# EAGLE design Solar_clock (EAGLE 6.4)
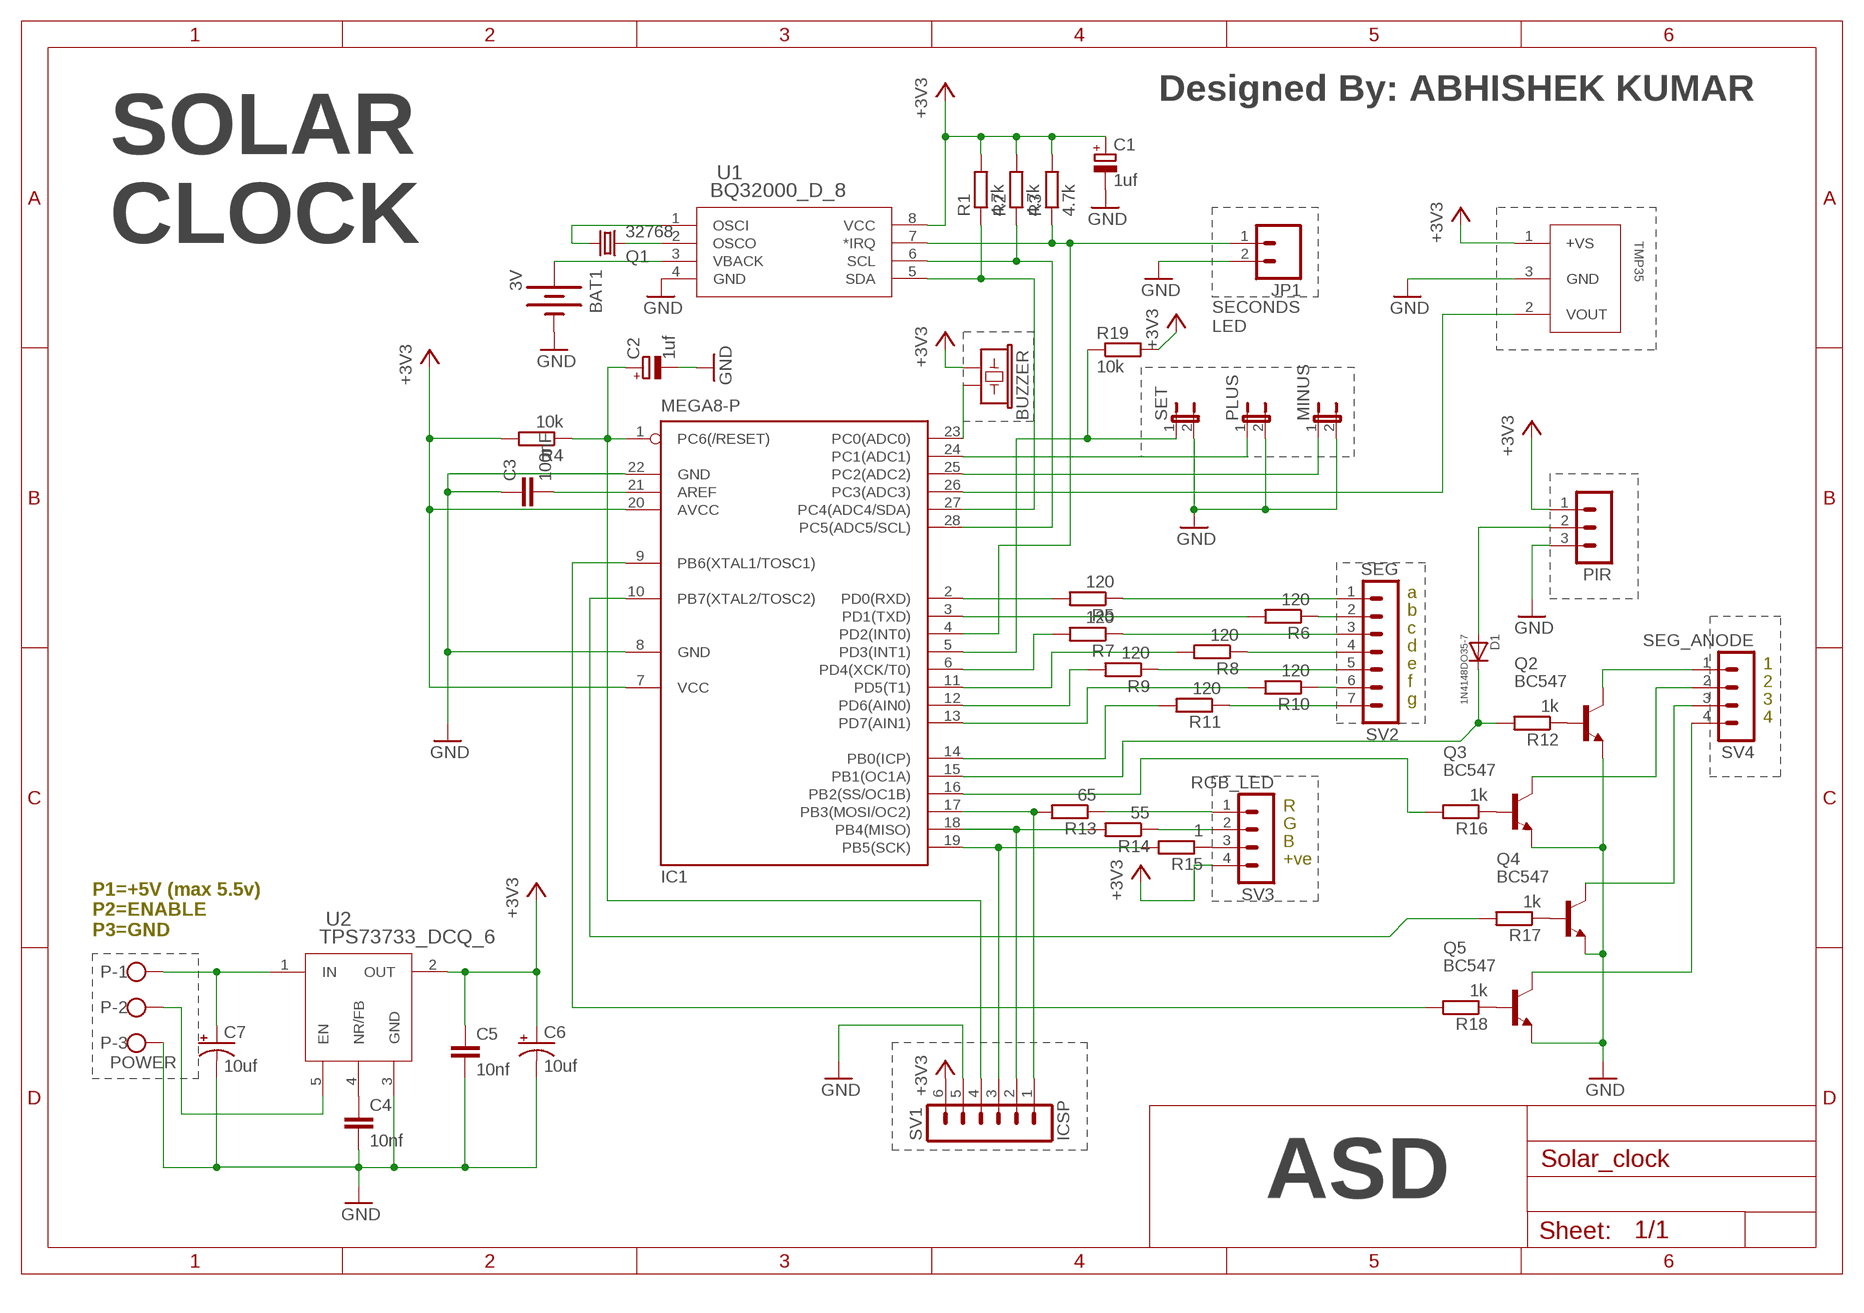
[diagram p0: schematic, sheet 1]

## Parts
BAT1  3V  BATTERY20PTH  [BATTCOM_20MM_PTH]
BUZZER  BUZZERNS  [BUZZER-12MM-NS]
C1  1uf  CPOL-EUE2.5-5  [E2,5-5]
C2  1uf  CPOL-EUE5-5  [E5-5]
C3  100nF  C-EU050-024X044  [C050-024X044]
C4  10nf  C-EU050-030X075  [C050-030X075]
C5  10nf  C-EU050-025X075  [C050-025X075]
C6  10uf  CPOL-USE2.5-6  [E2,5-6]
C7  10uf  CPOL-USE2.5-6  [E2,5-6]
D1  1N4148DO35-7  [DO35-7]
IC1  MEGA8-P  [DIL28-3]
JP1  M02PTH  [1X02]
MINUS  JUMPER-2PTH  [1X02]
P  POWER  W237-103  [W237-103]
PIR  MA03-1  [MA03-1]
PLUS  JUMPER-2PTH  [1X02]
Q1  32768  CRYSTALTC38H  [TC38H]
Q2  BC547  [TO92]
Q3  BC547  [TO92]
Q4  BC547  [TO92]
Q5  BC547  [TO92]
R1  4.7k  R-EU_R1206  [R1206]
R2  4.7k  R-EU_R1206  [R1206]
R3  4.7k  R-EU_R1206  [R1206]
R4  10k  R-EU_R1206  [R1206]
R5  120  R-EU_R1206  [R1206]
R6  120  R-EU_R1206  [R1206]
R7  120  R-EU_R1206  [R1206]
R8  120  R-EU_R1206  [R1206]
R9  120  R-EU_R1206  [R1206]
R10  120  R-EU_R1206  [R1206]
R11  120  R-EU_R1206  [R1206]
R12  1k  R-EU_R1206  [R1206]
R13  65  R-EU_R1206  [R1206]
R14  55  R-EU_R1206  [R1206]
R15  1  R-EU_R1206  [R1206]
R16  1k  R-EU_R1206  [R1206]
R17  1k  R-EU_R1206  [R1206]
R18  1k  R-EU_R1206  [R1206]
R19  10k  R-EU_R1206  [R1206]
SET  JUMPER-2PTH  [1X02]
SV1  ICSP  MA06-1  [MA06-1]
SV2  SEG  MA07-1  [MA07-1]
SV3  RGB_LED  MA04-1  [MA04-1]
SV4  SEG_ANODE  MA04-1  [MA04-1]
TMP35  TMP35GT9  [T_3]
U1  BQ32000_D_8  [D8]
U2  TPS73733_DCQ_6  [DCQ6]

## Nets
+3V3: BUZZER.+ C1.+ C5.1 C6.+ IC1.7(VCC) IC1.20(AVCC) PIR.1 R1.2 R2.2 R3.2 R4.2 R19.2 SV1.6 SV3.4 TMP35.1(+VS) U1.8(VCC) U2.2(OUT)
GND: BAT1.2(-) C1.- C2.- C3.1 C4.2 C5.2 C6.- C7.- IC1.8(GND) IC1.22(GND) JP1.2 MINUS.2 P.3 PIR.3 PLUS.2 Q2.1(E) Q3.1(E) Q4.1(E) Q5.1(E) SET.2 SV1.5 TMP35.3(GND) U1.4(GND) U2.3(GND)
N$1: IC1.28(PC5(ADC5/SCL)) R2.1 U1.6(SCL)
N$2: IC1.27(PC4(ADC4/SDA)) R1.1 U1.5(SDA)
N$3: IC1.4(PD2(INT0)) JP1.1 R3.1 U1.7(*IRQ)
N$4: Q1.2 U1.2(OSCO)
N$5: Q1.1 U1.1(OSCI)
N$6: C2.+ IC1.1(PC6(/RESET)) R4.1 SV1.4
N$7: C3.2 IC1.21(AREF)
N$8: IC1.17(PB3(MOSI/OC2)) R13.2 SV1.1
N$9: IC1.18(PB4(MISO)) R14.2 SV1.2
N$10: IC1.19(PB5(SCK)) R15.2 SV1.3
N$11: IC1.2(PD0(RXD)) R5.2
N$12: IC1.14(PB0(ICP)) R11.2
N$13: IC1.13(PD7(AIN1)) R10.2
N$14: IC1.6(PD4(XCK/T0)) R7.2
N$15: IC1.11(PD5(T1)) R8.2
N$16: R15.1 SV3.3
N$17: IC1.3(PD1(TXD)) R6.2
N$18: IC1.12(PD6(AIN0)) R9.2
N$19: IC1.5(PD3(INT1)) R19.1 SET.1
N$20: IC1.24(PC1(ADC1)) PLUS.1
N$21: IC1.25(PC2(ADC2)) MINUS.1
N$22: IC1.26(PC3(ADC3)) TMP35.2(VOUT)
N$23: BUZZER.- IC1.23(PC0(ADC0))
N$24: R5.1 SV2.1
N$25: R6.1 SV2.2
N$26: R7.1 SV2.3
N$27: R10.1 SV2.6
N$28: R9.1 SV2.5
N$29: R11.1 SV2.7
N$30: R8.1 SV2.4
N$31: R14.1 SV3.2
N$32: R13.1 SV3.1
N$33: Q2.2(B) R12.1
N$34: Q3.2(B) R16.1
N$35: Q4.2(B) R17.1
N$36: Q5.2(B) R18.1
N$37: Q3.3(C) SV4.2
N$38: Q5.3(C) SV4.4
N$39: Q4.3(C) SV4.3
N$40: Q2.3(C) SV4.1
N$41: D1.C IC1.15(PB1(OC1A)) R12.2
N$42: IC1.16(PB2(SS/OC1B)) R16.2
N$43: IC1.10(PB7(XTAL2/TOSC2)) R17.2
N$44: IC1.9(PB6(XTAL1/TOSC1)) R18.2
N$45: BAT1.1(+) U1.3(VBACK)
N$46: C4.1 U2.4(NR/FB)
N$47: C7.+ P.1 U2.1(IN)
N$48: P.2 U2.5(EN)
N$51: D1.A PIR.2

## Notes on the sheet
- Designed By: ABHISHEK KUMAR
- SOLAR
- CLOCK
- SECONDS
  LED
- a
- b
- c
- d
- e | 1
- f | 2
- g | 3
- 4
- R
- G
- B
- +ve
- P1=+5V (max 5.5v)
  P2=ENABLE
  P3=GND
- ASD

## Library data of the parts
BAT1 = SparkFun:BATTERY: Battery Holders
BUZZER = SparkFun:BUZZER: Buzzer 12mm
C1 C2 = resistor:CPOL-EU: POLARIZED CAPACITOR, European symbol
C3-C5 = resistor:C-EU: CAPACITOR, European symbol
C6 C7 = resistor:CPOL-US: POLARIZED CAPACITOR, American symbol
D1 = diode:1N4148: DIODE
IC1 = atmel:MEGA8-P: MICROCONTROLLER 8 Kbytes FLASH, 1 kbytes SRAM, 512 bytes EEPROM, USART, 4-channel 10 bit ADC, 2-channel 8 bit ADC Pin compatible with Atmega48, ATMega88, ATMega168 Source: avr.lbr; OC_FARNELL: unknown; OC_NEWARK: unknown
JP1 = SparkFun:M02: Header 2
MINUS PLUS SET = SparkFun:JUMPER-2: Jumper
P = con-wago-500:W237-103: WAGO SCREW CLAMP; MPN: 237-103; OC_FARNELL: unknown; OC_NEWARK: 18M7116
PIR = con-lstb:MA03-1: PIN HEADER; OC_FARNELL: unknown; OC_NEWARK: unknown
Q1 = SparkFun:CRYSTAL: Crystals
Q2-Q5 = transistor-npn:BC547*: NPN Transistor
R1-R19 = resistor:R-EU_: RESISTOR, European symbol
SV1 = con-lstb:MA06-1: PIN HEADER; OC_FARNELL: unknown; OC_NEWARK: unknown
SV2 = con-lstb:MA07-1: PIN HEADER; OC_FARNELL: unknown; OC_NEWARK: unknown
SV3 SV4 = con-lstb:MA04-1: PIN HEADER; OC_FARNELL: unknown; OC_NEWARK: unknown
TMP35 = TMP35:TMP35GT9; MANUFACTURER_PART_NUMBER: TMP35GT9; VENDOR: Vendor
U1 = BQ32000:BQ32000_D_8; DATASHEETURL: http://www.ti.com/lit/gpn/BQ32000; DESCRIPTION: Serial RTC with Battery Backup and Trickle Charge; FAMILY_NAME: REAL-TIME CLOCK; GENERIC_PART_NUMBER: BQ32000; INDUSTRY_STD_PKG_TYPE: SOIC; MANUFACTURER: Texas Instruments; PACKAGE_DESIGNATOR: D; PIN_COUNT: 8
U2 = TPS73733:TPS73733_DCQ_6; DATASHEETURL: http://www.ti.com/lit/gpn/TPS73733; DESCRIPTION: Single Output LDO, 1A, Fixed (3.3V), Reverse Current Protection; FAMILY_NAME: SINGLE CHANNEL LDO; GENERIC_PART_NUMBER: TPS73733; INDUSTRY_STD_PKG_TYPE: SOT-223; MANUFACTURER: Texas Instruments; MANUFACTURER_PART_NUMBER: tps73733_dcq_6; PACKAGE_DESIGNATOR: DCQ; PIN_COUNT: 6; VENDOR: Texas Instruments

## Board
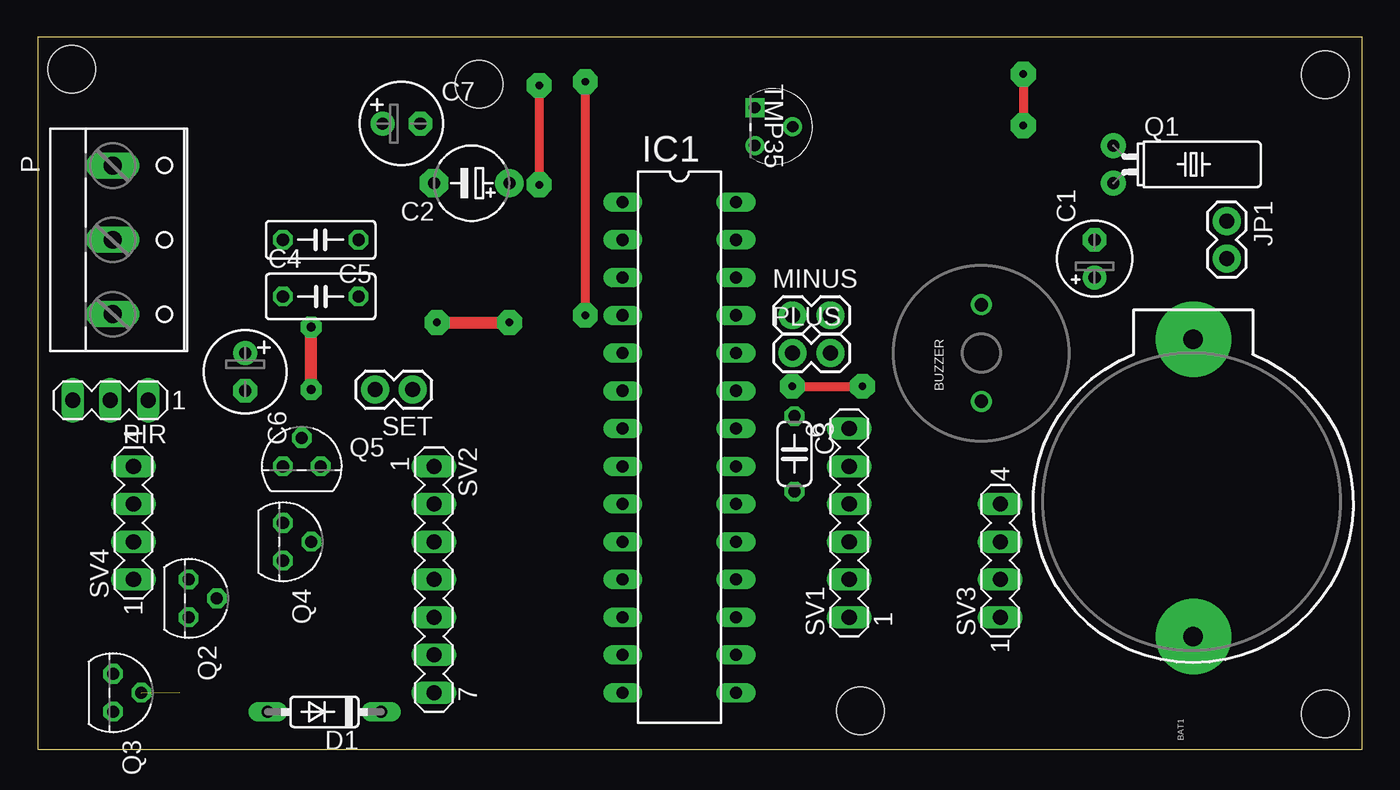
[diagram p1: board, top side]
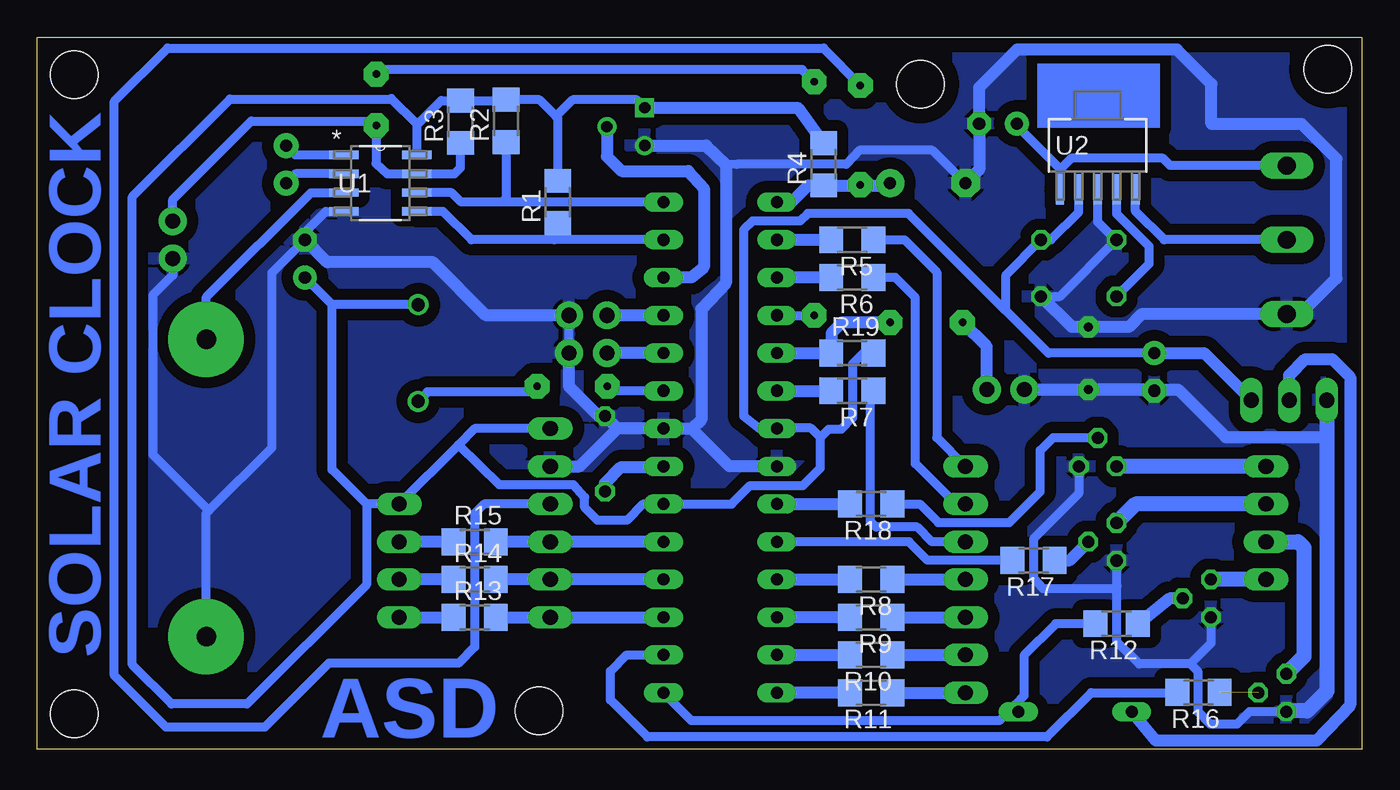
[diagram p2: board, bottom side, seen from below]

Size 89.13 x 47.93 mm. Coordinates in mm from the lower left corner, seen from the top.
Outline: 0,0 89.13,0 89.13,47.93 0,47.93 0,0
Copper layers (1*16): Top 0.035mm / dielectric 1.5mm / Bottom 0.035mm
Design rules "default *": minimum track width 10mil, minimum drill 24mil, track to track 30mil, track to pad 30mil, pad to pad 8mil, via to via 8mil, smd to smd 8mil, copper to edge 40mil, drill to drill 8mil, minimum pad ring 10mil, minimum via ring 8mil, stop-mask expansion 4mil, vias tented up to drill 0mil, thermal gap 10mil
Holes 3.2 mm at 86.64,45.42 86.64,2.39 29.72,44.75 2.29,45.77 55.37,2.59

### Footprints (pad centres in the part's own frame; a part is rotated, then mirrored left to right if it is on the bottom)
BATTCOM_20MM_PTH = drill 1.3: 1 20,0; 2 0,0
BUZZER-12MM-NS = drill 0.9: + 3.25,0; - -3.25,0
E2,5-5 = drill 0.813 pad 1.6: + -1.27,0 | drill 0.813 pad 1.6 octagon: - 1.27,0
E5-5 = drill 0.813 pad 1.905: + -2.54,0 | drill 0.813 pad 1.905 octagon: - 2.54,0
C050-024X044 = drill 0.813 octagon: 1 -2.54,0; 2 2.54,0
C050-030X075 = drill 0.813 octagon: 1 -2.54,0; 2 2.54,0
C050-025X075 = drill 0.813 octagon: 1 -2.54,0; 2 2.54,0
E2,5-6 = drill 0.813 pad 1.6: + -1.27,0 | drill 0.813 pad 1.6 octagon: - 1.27,0
DO35-7 = drill 0.813 long: A 3.81,0; C -3.81,0
DIL28-3 = drill 0.813 long: 1 -16.51,-3.81; 2 -13.97,-3.81; 3 -11.43,-3.81; 4 -8.89,-3.81; 5 -6.35,-3.81; 6 -3.81,-3.81; 7 -1.27,-3.81; 8 1.27,-3.81; 9 3.81,-3.81; 10 6.35,-3.81; 11 8.89,-3.81; 12 11.43,-3.81; 13 13.97,-3.81; 14 16.51,-3.81; 15 16.51,3.81; 16 13.97,3.81; 17 11.43,3.81; 18 8.89,3.81; 19 6.35,3.81; 20 3.81,3.81; 21 1.27,3.81; 22 -1.27,3.81; 23 -3.81,3.81; 24 -6.35,3.81; 25 -8.89,3.81; 26 -11.43,3.81; 27 -13.97,3.81; 28 -16.51,3.81
1X02 = drill 1.016 pad 1.88: 1 0,0; 2 2.54,0
W237-103 = drill 1.194 long: 1 -5,-1.29; 2 0,-1.29; 3 5,-1.29
MA03-1 = drill 1.016 long: 1 -2.54,0; 2 0,0; 3 2.54,0
TC38H = drill 0.813 pad 1.676: 1 -1.27,0; 2 1.27,0
TO92 = drill 0.813 octagon: 1 1.27,0; 2 0,1.905; 3 -1.27,0
R1206 = smd 1.6 x 1.803: 1 -1.422,0; 2 1.422,0
MA06-1 = drill 1.016 long: 1 -6.35,0; 2 -3.81,0; 3 -1.27,0; 4 1.27,0; 5 3.81,0; 6 6.35,0
MA07-1 = drill 1.016 long: 1 -7.62,0; 2 -5.08,0; 3 -2.54,0; 4 0,0; 5 2.54,0; 6 5.08,0; 7 7.62,0
MA04-1 = drill 1.016 long: 1 -3.81,0; 2 -1.27,0; 3 1.27,0; 4 3.81,0
T_3 = drill 0.762 square: 1 -2.54,-2.54 | drill 0.762: 2 -1.27,0; 3 0,-2.54
D8 = smd 1.981 x 0.559: 1 -2.464,1.905; 2 -2.464,0.635; 3 -2.464,-0.635; 4 -2.464,-1.905; 5 2.464,-1.905; 6 2.464,-0.635; 7 2.464,0.635; 8 2.464,1.905
DCQ6 = smd 0.559 x 2.057: 1 -2.54,-2.946; 2 -1.27,-2.946; 3 0,-2.946; 4 1.27,-2.946; 5 2.54,-2.946

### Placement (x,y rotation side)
BAT1  77.75,7.59 90 top
BUZZER  63.5,26.67 90 top
C1  71.12,33.02 90 top
C2  29.21,38.1 180 top
C3  50.93,19.89 270 top
C4  19.05,30.48 0 top
C5  19.05,34.29 180 top
C6  13.97,25.4 270 top
C7  24.49,42.11 0 top
D1  19.3,2.51 180 top
IC1  43.18,20.32 270 top
JP1  80.01,35.56 270 top
MINUS  50.8,29.21 0 top
P  6.35,34.29 270 top
PIR  4.9,23.5 180 top
PLUS  50.8,26.67 0 top
Q1  72.39,39.37 270 top
Q2  10.16,10.16 270 top
Q3  5.08,3.81 270 top
Q4  16.51,13.97 270 top
Q5  17.78,19.05 0 top
R1  54.1,36.83 90 bottom
R2  57.58,42.29 90 bottom
R3  60.66,42.24 90 bottom
R4  36.22,39.37 90 bottom
R5  34.29,34.29 180 bottom
R6  34.29,31.75 180 bottom
R7  34.29,24.13 180 bottom
R8  33.02,11.43 180 bottom
R9  33.02,8.89 180 bottom
R10  33.02,6.35 180 bottom
R11  33.02,3.81 180 bottom
R12  16.51,8.46 180 bottom
R13  59.69,8.89 0 bottom
R14  59.69,11.43 0 bottom
R15  59.69,13.97 0 bottom
R16  11,3.84 180 bottom
R17  22.1,12.73 180 bottom
R18  33.02,16.51 180 bottom
R19  34.29,26.67 0 bottom
SET  25.25,24.21 180 top
SV1  54.61,15.24 90 top
SV2  26.67,11.43 270 top
SV3  64.77,12.7 90 top
SV4  6.45,15.24 90 top
TMP35  50.8,40.64 270 top
U1  66.04,38.1 0 bottom
U2  17.78,40.64 0 bottom

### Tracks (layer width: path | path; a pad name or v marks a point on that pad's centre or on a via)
+3V3
  Bottom 0.61: TMP35.1 48.79,43.71 53.11,43.71 54.23,42.6 | R1.2 54.1,42.47 54.23,42.6 | 54.23,42.6 55.35,43.71 R2.2 57.63,43.66 R3.2 61.95,43.66 63.58,42.04 U1.8 63.58,42.06 65.3,43.79 65.33,43.76 76.15,43.76 82.73,37.19 82.73,5.69 80.09,3.05 75.01,3.05 66.98,11.07 66.98,16.51 | BUZZER.+ 69.29,29.92 | 69.29,29.92 C1.+ | 66.98,16.51 SV3.4 60.8,20.48 | 66.98,16.51 69.29,18.82 69.29,29.92 | SV1.6 59.69,21.59 60.8,20.48 | U2.2 19.05,36.17 20.93,34.29 C5.1 23.95,31.93 23.95,29.54 | C6.+ 21.08,26.67 23.95,29.54 | 36.45,20.98 36.45,18.92 37.62,17.75 41.17,17.75 42.42,16.51 IC1.20 48.36,16.51 49.45,15.42 51.44,15.42 52.3,16.28 52.3,16.97 53.06,17.81 58.04,17.81 60.8,20.48 | 36.45,20.98 37.08,21.61 39.35,21.61 IC1.7 39.4,21.56 40.51,21.56 41.61,22.43 41.61,34.98 41,35.56 37.8,35.56 37.29,36.07 30.5,36.07 23.98,29.54 23.95,29.54 | R19.2 33.53,26.67 34.27,25.93 34.27,22.33 35.05,21.54 35.89,21.54 36.45,20.98
  Bottom 0.813: TMP35.1 37.95,43.18 R4.2 | C6.+ 10.62,26.67 PIR.1
GND  (via drill 0.6 pad 1.42)
  Top 0.813: v18.41,24.21 v18.41,28.42
  Bottom 0.61: U1.4 69.72,36.2 71.12,34.8 C1.- 73.33,32.08 73.33,20.32 77.58,16.06 | PLUS.2 MINUS.2 | 53.67,19.05 SV1.5 | U2.3 17.78,35.48 16.59,34.29 C5.2 20.32,30.48 C4.2 20.62,30.48 | Q3.1 7.57,2.54 8.41,1.7 10.21,1.7 11.02,2.52 11.02,5.21 11.56,5.74 | 11.56,5.74 14.99,5.74 16.48,7.24 16.48,10.97 | 16.48,10.97 16.48,12.67 Q4.1 | Q2.1 10.16,7.14 11.56,5.74 | Q5.1 19.05,17.22 22.1,14.15 22.1,11.53 21.46,10.82 16.64,10.82 16.48,10.97 | C2.- 26.69,38.1 28.9,40.31 33.81,40.31 34.7,39.37 42.06,39.37 42.8,39.34 | BAT1.2 77.75,15.9 77.58,16.06 | JP1.2 80.01,31.9 81.36,30.56 81.36,19.84 77.58,16.06
  Bottom 0.813: TMP35.3 44.12,40.64 42.8,39.34 42.8,31.39 44.45,29.64 44.45,22.17 45.06,21.56 | C2.- 25.76,39.01 C7.- 25.76,44.55 23.22,47.09 12.45,47.09 10.13,44.78 10.13,42.09 4.06,42.09 1.73,39.75 1.73,31.7 4.14,29.29 P.3 14.83,29.29 15.7,28.42 v18.41,28.42 19.53,28.42 C4.2 | 45.06,21.56 46.97,21.56 IC1.22 50.09,21.59 | IC1.8 42.55,19.05 45.06,21.56 | 50.09,21.59 C3.1 51.36,22.43 53.34,24.41 PLUS.2 | 53.67,19.05 52.63,19.05 50.09,21.59 | MINUS.2 58.93,29.21 62.51,32.79 69.62,32.79 C1.- | SET.2 v18.41,24.21 | C6.- 14.05,24.21 v18.41,24.21 | v18.41,24.21 12.37,24.21 9.17,21.01 2.69,21.01 2.36,20.68
  Bottom 1.016: PIR.3 2.36,20.68 2.36,3.91 3.68,2.59 5.03,2.59 Q3.1
  pour Bottom: -0.03,47.98 -0.03,0 89.1,-0.25 89.1,47.7 0.97,47.98
N$1
  Bottom 0.61: IC1.28 57.86,36.83 | 57.86,36.83 60.6,36.83 61.24,37.47 U1.6 | R2.1 57.58,37.11 57.86,36.83
N$2
  Bottom 0.61: IC1.27 54.33,34.29 | 54.33,34.29 59.92,34.29 61.82,36.2 U1.5 | R1.1 54.1,34.52 54.33,34.29
N$3  (via drill 0.5 pad 1.68)
  Top 0.61: v36.86,29.21 v36.86,44.93 | v66.32,45.44 v66.32,41.99
  Bottom 0.61: R3.1 60.66,39.14 61.06,38.73 U1.7 65.58,38.73 66.34,39.42 66.34,41.63 v66.32,41.99 66.62,42.29 74.73,42.29 80.01,37.01 JP1.1 | IC1.4 v36.86,29.21 | v36.86,44.93 37.67,45.75 66.02,45.75 v66.32,45.44
N$4
  Bottom 0.61: U1.2 71.75,38.73 Q1.2
N$5
  Bottom 0.61: U1.1 71.75,40 Q1.1
N$6  (via drill 0.5 pad 1.68)
  Top 0.61: v33.76,44.68 v33.76,38
  Bottom 0.61: SV1.4 59.05,16.51 59.69,15.88 59.69,6.88 60.78,5.79 69.52,5.79 73.81,1.5 80.47,1.5 83.95,4.98 83.95,43.61 80.37,47.19 36.22,47.19 v33.76,44.68 | v33.76,38 33.53,37.95
  Bottom 0.813: IC1.1 38.38,36.83 37.26,37.95 35.56,37.95 R4.1 33.53,37.95 31.9,37.95 C2.+
N$7
  Bottom 0.813: C3.2 50.93,17.91 49.84,19 47.04,19 IC1.21
N$8
  Bottom 0.813: R13.2 SV1.1 IC1.17
N$9
  Bottom 0.813: IC1.18 SV1.2 R14.2
N$10
  Bottom 0.813: IC1.19 SV1.3 R15.2
N$11
  Bottom 0.813: IC1.2 R5.2
N$12
  Bottom 0.813: R11.2 IC1.14
N$13
  Bottom 0.813: IC1.13 R10.2
N$14
  Bottom 0.813: IC1.6 R7.2
N$15
  Bottom 0.813: IC1.11 R8.2
N$16
  Bottom 0.813: R15.1 SV3.3
N$17
  Bottom 0.813: R6.2 IC1.3
N$18
  Bottom 0.813: R9.2 IC1.12
N$19  (via drill 0.5 pad 1.68)
  Top 0.813: v26.87,28.73 v31.75,28.73
  Bottom 0.813: IC1.5 R19.1 35.69,26.7 35.69,28.02 34.98,28.73 v31.75,28.73 | SET.1 25.25,27.1 v26.87,28.73
N$20
  Bottom 0.813: IC1.24 PLUS.1
N$21
  Bottom 0.813: IC1.25 MINUS.1
N$22
  Bottom 0.813: TMP35.2 50.8,39.9 49.81,38.91 45.34,38.91 44.27,37.74 44.27,32.46 45.14,31.75 IC1.26
N$23  (via drill 0.5 pad 1.68)
  Top 0.61: v50.78,24.44 v55.5,24.44
  Bottom 0.61: IC1.23 50.29,24.13 v50.78,24.44 | v55.5,24.44 55.88,24.05 62.87,24.05 BUZZER.-
N$24
  Bottom 0.61: R5.1 30.79,34.29 28.6,32.11 28.6,20.98 SV2.1
N$25
  Bottom 0.61: SV2.2 27.33,16.51 30.05,19.23 30.05,30.4 31.39,31.75 R6.1
N$26
  Bottom 0.61: SV2.3 28.93,13.97 29.92,14.96 32.69,14.96 33.07,15.34 33.07,23.93 R7.1
N$27
  Bottom 0.813: R10.1 SV2.6
N$28
  Bottom 0.813: R9.1 SV2.5
N$29
  Bottom 0.813: R11.1 SV2.7
N$30
  Bottom 0.813: R8.1 SV2.4
N$31
  Bottom 0.813: R14.1 SV3.2
N$32
  Bottom 0.813: SV3.1 R13.1
N$33
  Bottom 0.813: Q2.2 12.95,10.16 R12.1
N$34  (1 unrouted)
N$35
  Bottom 0.813: R17.1 19.66,12.72 Q4.2
N$36
  Bottom 0.61: R18.1 29.74,16.51 28.5,15.27 23.72,15.27 21.64,17.35 21.64,20.12 20.78,20.98 17.8,20.98 Q5.2
N$37
  Bottom 1.016: SV4.2 4.29,13.97 3.91,13.59 3.91,6.25 Q3.3
N$38
  Bottom 1.016: SV4.4 Q5.3
N$39
  Bottom 1.016: SV4.3 15.24,16.51 Q4.3
N$40
  Bottom 1.016: SV4.1 Q2.3
N$41
  Bottom 0.61: R12.2 20.6,8.46 22.73,6.33 22.73,3.61 23.33,3.01 | 23.33,3.01 24.41,1.93 45.11,1.93 IC1.15 | D1.C 23.11,2.79 23.33,3.01
N$42
  Bottom 0.61: IC1.16 49.48,6.35 50.57,5.26 50.57,3.33 48.08,0.84 21.18,0.84 18.21,3.81 12.45,3.81 R16.2
N$43
  Bottom 0.61: R17.2 29.23,12.72 30.48,13.97 IC1.10
N$44
  Bottom 0.813: IC1.9 R18.2
N$45
  Bottom 0.61: BAT1.1 77.75,30.43 70.71,37.47 U1.3
N$46
  Bottom 0.61: U2.4 16.51,36.04 14.33,33.86 14.33,32.66 C4.1
N$47
  Bottom 0.61: P.1 12.9,39.29 13.39,39.78 19.56,39.78 20.29,39.04 | 20.29,39.04 20.29,37.72 U2.1 | C7.+ 23.22,41.96 20.29,39.04
N$48
  Bottom 0.61: P.2 13.31,34.29 15.24,36.22 U2.5
N$49  (via drill 0.5 pad 5.08)
  other vias: 77.77,27.61
N$50  (via drill 0.5 pad 5.08)
  other vias: 77.77,7.59
N$51
  Bottom 0.813: D1.A 13.87,0.58 3.07,0.58 0.79,2.97 0.79,25.04 2.01,26.26 3.81,26.26 4.9,25.17 PIR.2
(copper drawn outside any net)
  shapes: Bottom area x1

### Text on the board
Bottom: SOLAR CLOCK | ASD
